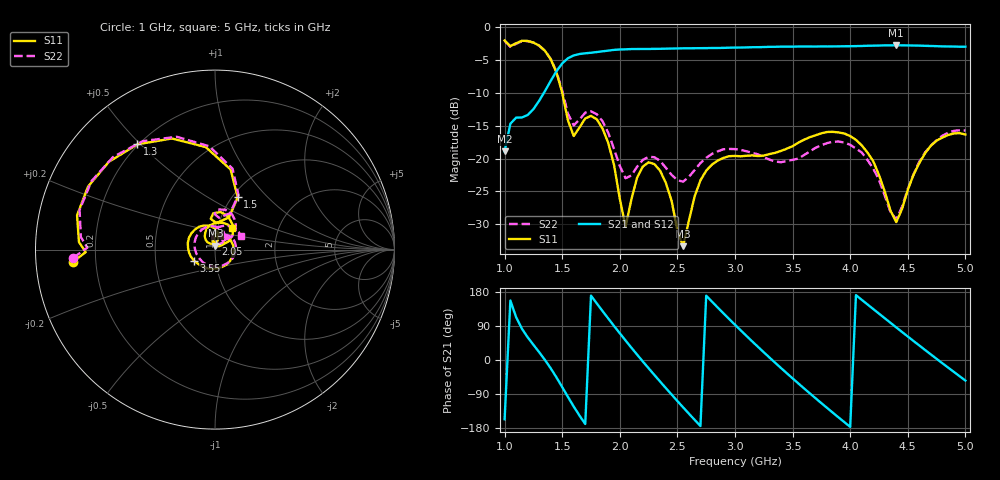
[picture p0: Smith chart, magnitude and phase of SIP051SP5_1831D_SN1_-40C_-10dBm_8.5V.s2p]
# GHz  S  dB  R  50
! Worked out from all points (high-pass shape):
!   81 points, 1 GHz to 5 GHz, reference 50 ohm
!   highest |S21| = -2.71 dB at 4.4 GHz (marker M1); lowest = -18.9 dB at 1 GHz (marker M2)
!   |S21| within 3 dB of the highest: 1.49 GHz to end of sweep
!   lowest |S11| = -33.4 dB at 2.55 GHz (marker M3), VSWR 1.04, Z = 50.2 + j2.14 ohm
!   |S11| at or under -10 dB: 1.5 GHz to end of sweep
!   |S22| runs from -29.3 to -2.0 dB; largest |S21 - S12| = 0.0026
!   S11 on the Smith chart (normalised r, x): 1 GHz: 0.11, -0.04; 1.3 GHz: 0.20, +0.49; 1.5 GHz: 1.06, +0.69; 2.05 GHz: 1.01, +0.06; 3.55 GHz: 0.78, -0.10; 5 GHz: 1.16, +0.29
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1  -1.98 -174.9  -18.90 -156.4  -18.92 -156.2  -2.03 -176.7
1.1  -2.40 176.9  -13.75 112.9  -13.76 113.0  -2.49 174.7
1.3  -2.75 126.4  -11.17 20.7  -11.18 20.6  -2.78 123.7
1.5  -9.96 66.5  -5.48 -71.5  -5.47 -71.4  -9.63 66.7
1.6  -16.55 86.7  -4.26 -122.7  -4.25 -122.7  -14.93 83.0
1.7  -13.88 92.8  -3.94 -169.0  -3.94 -168.9  -13.00 85.6
1.9  -17.64 41.0  -3.53 109.4  -3.52 109.5  -16.07 43.4
2.05  -30.39 77.5  -3.33 51.5  -3.33 51.5  -22.99 54.0
2.2  -21.21 91.0  -3.27 -4.0  -3.28 -3.9  -20.20 68.1
2.35  -21.85 52.7  -3.25 -56.9  -3.24 -56.9  -20.35 49.0
2.55  -33.36 82.8  -3.17 -125.1  -3.17 -125.0  -23.52 54.3
2.75  -21.84 77.1  -3.14 169.7  -3.14 169.9  -19.88 52.8
3  -19.59 -3.2  -3.06 92.9  -3.06 92.9  -18.55 10.4
3.3  -19.31 -95.7  -2.95 6.3  -2.96 6.3  -20.17 -63.4
3.55  -17.57 -152.7  -2.90 -61.8  -2.90 -61.9  -20.00 -150.3
3.7  -16.44 175.9  -2.90 -101.1  -2.90 -101.1  -18.35 160.7
4  -16.57 115.4  -2.86 -176.5  -2.86 -176.6  -17.90 86.1
4.15  -19.08 86.9  -2.79 146.7  -2.78 146.7  -20.21 56.4
4.35  -27.95 79.7  -2.73 98.1  -2.74 98.2  -28.16 52.4
4.4  -29.69 102.6  -2.71 86.0  -2.71 86.0  -29.28 75.9
4.7  -18.04 111.3  -2.82 14.7  -2.82 14.8  -18.03 81.5
5  -16.33 52.8  -2.93 -54.3  -2.94 -54.4  -15.70 26.5
